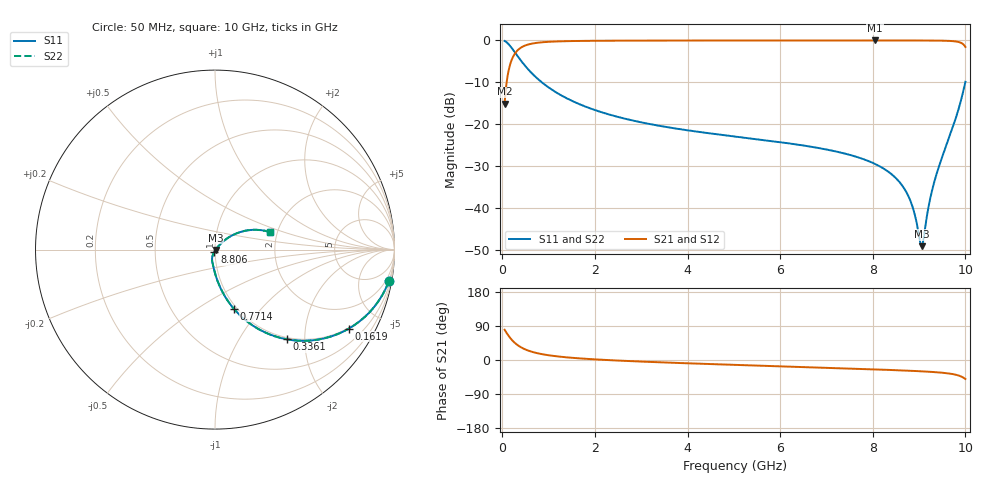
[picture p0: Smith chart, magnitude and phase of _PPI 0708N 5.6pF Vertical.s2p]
! S-Parameter data specifications (vertical orientation):
! Substrate: 40-mil Rogers 3003C, Substrate thickness, H=1.016mm, Dielectric constant, Er=3, Conductor thickness, T_mtl=0.043mm, Loss Tangent, Tand=0.003
! PCB Mounting Pad Footprint: Pad width, PadW=2.54mm , Pad length, PadL=0.51mm , Pad gap, PadG (edge-to-edge)=0.71mm , Reference planes=1.73mm apart
! Created Tue Jan 16 08:45:57 2018
# GHz S MA R 50
! 2 Port Network Data from SP1.SP block
! freq  magS11  angS11  magS21  angS21  magS12  angS12  magS22  angS22
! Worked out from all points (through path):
!   801 points, 50 MHz to 10 GHz, reference 50 ohm
!   highest |S21| = -0.02 dB at 8.047 GHz (marker M1); lowest = -15.1 dB at 50 MHz (marker M2)
!   group delay of S21, straight-line fit = 16.7 ps
!   lowest |S11| = -49.1 dB at 9.055 GHz (marker M3), VSWR 1.01, Z = 50.3 - j0.197 ohm
!   |S11| at or under -10 dB: 852.6 MHz to 9.998 GHz (9.145 GHz wide, 169 % of centre)
!   |S22| runs from -49.1 to -0.1 dB; largest |S21 - S12| = 0
!   S11 on the Smith chart (normalised r, x): 50 MHz: 1, -11; 161.9 MHz: 0.97, -3.41; 336.1 MHz: 0.97, -1.65; 771.4 MHz: 0.97, -0.72; 8.806 GHz: 0.99, -0.02; 10 GHz: 1.82, +0.40
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0.05  0.9845 -10.3  0.1752 79.7  0.1752 79.7  0.9845 -10.3
0.1619375  0.8664 -30.5  0.4991 59.5  0.4991 59.5  0.8664 -30.5
0.2365625  0.7652 -40.9  0.6435 49.1  0.6435 49.1  0.7652 -40.9
0.3360625  0.642 -51.2  0.7663 38.8  0.7663 38.8  0.642 -51.2
0.522625  0.4751 -63.4  0.8796 26.6  0.8796 26.6  0.4751 -63.4
0.771375  0.3451 -72.4  0.9381 17.6  0.9381 17.6  0.3451 -72.4
1.716625  0.1688 -85.9  0.985 3.9  0.985 3.9  0.1688 -85.9
3.370812  0.09613 -95.4  0.9944 -5.9  0.9944 -5.9  0.09613 -95.4
5.025  0.07128 -102.0  0.9962 -12.9  0.9962 -12.9  0.07128 -102.0
6.691625  0.05359 -107.9  0.9969 -19.3  0.9969 -19.3  0.05359 -107.9
8.047313  0.0336 -111.6  0.9972 -24.8  0.9972 -24.8  0.0336 -111.6
8.345812  0.02686 -111.7  0.9972 -26.2  0.9972 -26.2  0.02686 -111.7
8.619438  0.01906 -110.1  0.997 -27.5  0.997 -27.5  0.01906 -110.1
8.806  0.01245 -105.6  0.9968 -28.4  0.9968 -28.4  0.01245 -105.6
8.9055  0.008425 -98.1  0.9966 -29.0  0.9966 -29.0  0.008425 -98.1
9.017437  0.004079 -64.2  0.9963 -29.7  0.9963 -29.7  0.004079 -64.2
9.05475  0.003509 -33.9  0.9961 -29.9  0.9961 -29.9  0.003509 -33.9
9.092063  0.004141 -2.1  0.996 -30.1  0.996 -30.1  0.004141 -2.1
9.216437  0.01122 36.4  0.9952 -31.0  0.9952 -31.0  0.01122 36.4
9.340813  0.02172 43.8  0.9941 -32.0  0.9941 -32.0  0.02172 43.8
9.776125  0.1106 40.9  0.9731 -38.4  0.9731 -38.4  0.1106 40.9
10  0.3201 17.8  0.8342 -50.1  0.8342 -50.1  0.3201 17.8
